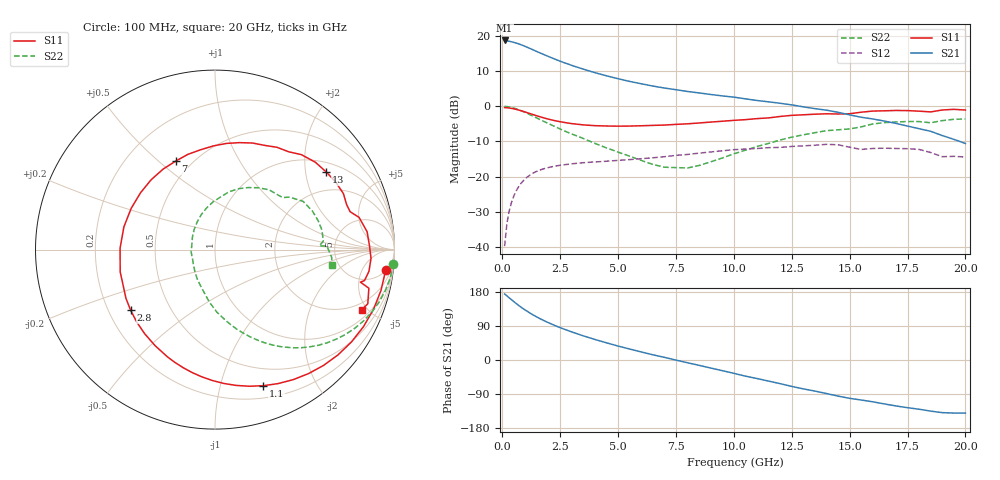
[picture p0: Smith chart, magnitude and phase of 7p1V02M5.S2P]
! Infineon Technologies  Discrete & RF Semiconductors
! bfp620
! VCE =  1.0 V,  IC =  2.5 mA
! Common Emitter S-Parameters:  Sep 2002
# GHz  S  MA  R  50
!  f  S11  S21  S12  S22
! GHz  MAG  ANG  MAG  ANG  MAG  ANG  MAG  ANG
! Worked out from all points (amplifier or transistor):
!   59 points, 100 MHz to 20 GHz, reference 50 ohm
!   highest |S21| = 18.7 dB at 100 MHz (marker M1)
!   |S21| within 3 dB of that: start of sweep to 1.44 GHz
!   unconditionally stable (mu >= 1): 5.625 GHz to 13.33 GHz; 14.26 GHz to 15.73 GHz; 17.16 GHz to end of sweep
!   at 1 GHz: K = 0.19, MSG = 18.8 dB, |S12| = -20.6 dB
!   at 5.5 GHz: K = 0.99, MSG = 11.1 dB, |S12| = -15.2 dB
!   at 20 GHz: K = 1.58, MAG = -2.6 dB, |S12| = -14.5 dB
!   S11 on the Smith chart (normalised r, x): 100 MHz: 5, -15; 1.1 GHz: 0.32, -1.37; 2.8 GHz: 0.29, -0.30; 7 GHz: 0.41, +0.57; 13 GHz: 1.29, +2.60; 20 GHz: 1.50, -4.58
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0.1  0.9577 -6.9  8.63 174.1  0.0102 83.9  0.9967 -4.5
0.3  0.9437 -20.6  8.4 164.0  0.0325 78.6  0.9774 -13.3
0.6  0.902 -40.6  7.922 149.0  0.0624 67.0  0.9182 -25.6
0.8  0.8652 -53.0  7.521 139.9  0.0792 59.8  0.8674 -33.0
1.1  0.8049 -70.4  6.85 127.6  0.0996 50.2  0.7845 -42.8
1.3  0.7657 -81.2  6.406 120.1  0.1103 44.7  0.7295 -48.5
1.5  0.7293 -91.2  5.989 113.2  0.119 39.9  0.6774 -53.5
1.9  0.6672 -109.5  5.258 101.0  0.1318 32.0  0.5855 -62.2
2.4  0.6109 -129.9  4.501 87.8  0.1428 24.2  0.4914 -71.3
2.8  0.5787 -144.3  4.029 78.6  0.1487 19.2  0.4286 -78.0
3.5  0.5426 -166.8  3.371 63.7  0.1572 12.0  0.3477 -88.4
4  0.5289 179.1  3.003 54.2  0.161 7.7  0.2959 -95.8
5  0.5205 153.8  2.463 36.8  0.1695 1.4  0.2225 -110.2
6  0.5273 132.4  2.088 21.3  0.1792 -4.3  0.1695 -130.8
7  0.5395 114.0  1.816 7.0  0.1914 -9.3  0.1357 -157.0
9  0.5951 83.8  1.47 -21.2  0.2235 -22.3  0.1617 135.9
10.5  0.6442 64.2  1.274 -42.6  0.2459 -35.3  0.2368 101.3
13  0.7555 35.0  0.98 -76.2  0.2731 -56.3  0.3918 61.9
13.5  0.7706 29.3  0.924 -82.0  0.2785 -61.1  0.4202 55.1
15  0.7816 15.7  0.754 -101.1  0.2613 -81.0  0.4754 37.6
17  0.8706 -3.2  0.57 -121.2  0.2505 -91.9  0.5971 15.6
20  0.8831 -22.4  0.295 -140.1  0.1894 -110.9  0.6588 -7.6
